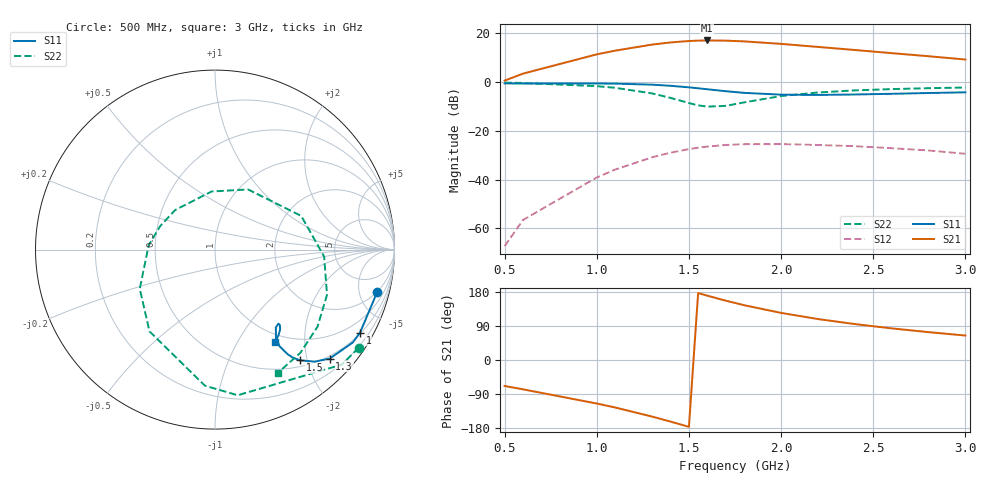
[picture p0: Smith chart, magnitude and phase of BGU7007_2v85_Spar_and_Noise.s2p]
! BGU7007, Vcc=2.85 V, Icc=5.2050 mA
# MHz S MA R 50
!  Freq-MHz  S11-mag  S11-arg  S21-mag  S21-arg  S12-mag  S12-arg  S22-mag  S22-arg
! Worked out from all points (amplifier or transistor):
!   17 points, 500 MHz to 3 GHz, reference 50 ohm
!   highest |S21| = 17.0 dB at 1.6 GHz (marker M1)
!   |S21| within 3 dB of that: 1.195 GHz to 2.256 GHz (1.061 GHz wide, 61.5 % of centre)
!   unconditionally stable (mu >= 1): start of sweep to 1.266 GHz; 1.775 GHz to end of sweep
!   at 1 GHz: K = 1.19, MAG = 22.6 dB, |S12| = -39.1 dB
!   at 1.6 GHz: K = 0.98, MSG = 21.7 dB, |S12| = -26.5 dB
!   at 3 GHz: K = 1.65, MAG = 14.6 dB, |S12| = -29.4 dB
!   S11 on the Smith chart (normalised r, x): 500 MHz: 2.01, -7.32; 1 GHz: 0.53, -3.69; 1.3 GHz: 0.45, -2.43; 1.5 GHz: 0.60, -1.87; 3 GHz: 0.88, -1.45
500  0.9336 -14.5  1.066 -68.6  0.0004345 -84.8  0.9698 -34.3
600  0.9292 -17.1  1.484 -77.4  0.001498 -94.1  0.954 -42.2
1000  0.9313 -29.8  3.682 -114.9  0.0111 -143.4  0.8214 -81.1
1100  0.9257 -34.0  4.381 -125.4  0.01611 -154.8  0.7603 -94.2
1300  0.8817 -43.5  5.83 -149.3  0.02865 -178.9  0.5838 -128.7
1400  0.8357 -48.3  6.456 -162.6  0.0356 167.3  0.4726 -152.5
1500  0.777 -52.5  6.9 -176.4  0.04222 153.2  0.3703 176.2
1550  0.7434 -54.2  7.025 176.6  0.04517 146.2  0.332 156.6
1600  0.7094 -55.2  7.085 169.7  0.04754 139.5  0.3129 135.2
1700  0.6472 -56.3  7.023 156.5  0.05137 126.3  0.3244 93.3
1800  0.5984 -55.4  6.782 144.6  0.05321 114.6  0.3824 61.2
2000  0.5506 -52.0  6.032 124.3  0.05351 95.0  0.5157 21.3
2200  0.5433 -49.4  5.223 108.0  0.05135 80.1  0.6093 -3.6
2400  0.5548 -49.4  4.519 94.8  0.04842 68.8  0.6731 -22.0
2600  0.5727 -50.7  3.896 83.5  0.04411 59.4  0.7149 -37.0
2800  0.5946 -53.5  3.369 73.5  0.03961 52.4  0.7463 -50.4
3000  0.6141 -57.2  2.885 64.5  0.03383 46.3  0.7701 -62.9
